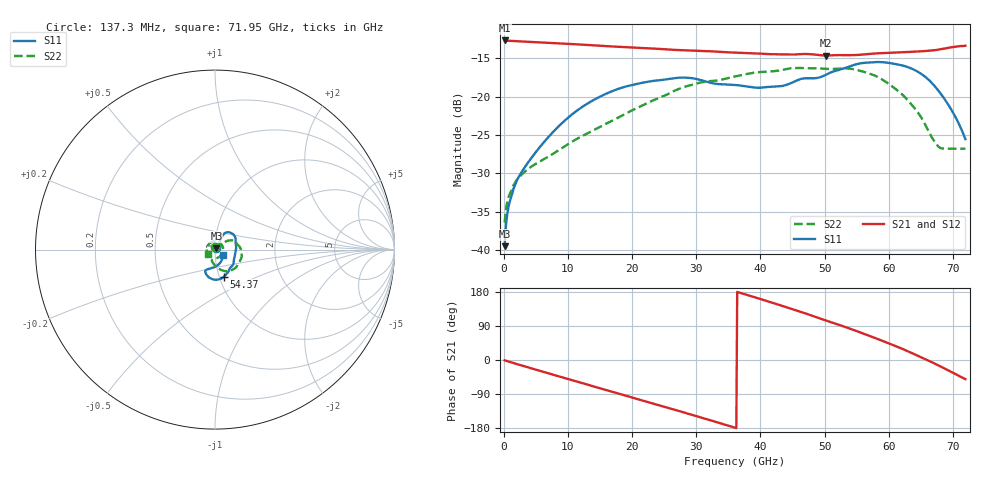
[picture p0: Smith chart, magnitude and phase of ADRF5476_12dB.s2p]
! Device:  ADRF5476
! Description: Flip-Chip, Silicon Digital Step Attenuator
! Frequency:  0.1 GHz -  72 GHz
! Ports:
!  RFC = ATTIN
!  RF1 = ATTOUT
! VDD  =  +3.3 Volts
! VSS  =  -3.3 Volts
! State
! 12dB Attenuation State: D0 = +3.3V, D1 = +3.3V
! Data:  Data was collected using a calibrated network analyzer
!  The reference plane is the package boundry of ADRF5476 switch.
! Notes: Analog Devices supplies this data as a sample of measured data
!  for this product.  Your particular data for this product may vary.
!  Analog Devices reserves the right to change this data at anytime.
# GHZ  S  DB  R  50
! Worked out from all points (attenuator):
!   524 points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, 137.3 MHz to 71.95 GHz, reference 50 ohm
!   highest |S21| = -12.67 dB at 137.3 MHz (marker M1); lowest = -14.6 dB at 50.26 GHz (marker M2)
!   lowest |S11| = -39.5 dB at 137.3 MHz (marker M3), VSWR 1.02, Z = 50.8 + j0.708 ohm
!   |S11| at or under -10 dB: start of sweep to end of sweep
!   |S22| runs from -36.4 to -16.3 dB; largest |S21 - S12| = 0.051
!   S11 on the Smith chart (normalised r, x): 137.3 MHz: 1.02, +0.01; 54.37 GHz: 1.05, -0.33; 71.95 GHz: 1.09, -0.07
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0.1373092  -39.48 41.0  -12.67 -0.9  -12.67 -0.9  -36.40 94.8
0.5492366  -35.29 42.7  -12.70 -3.0  -12.70 -3.0  -33.72 48.4
0.9611641  -33.61 41.9  -12.72 -5.2  -12.72 -5.2  -32.65 38.6
1.785019  -31.42 42.9  -12.76 -9.4  -12.75 -9.4  -31.17 25.0
2.608874  -30.07 44.5  -12.79 -13.5  -12.79 -13.5  -30.29 25.5
7.277386  -24.97 59.2  -12.99 -36.7  -12.98 -36.7  -27.65 32.9
12.22052  -21.34 61.9  -13.22 -61.0  -13.22 -61.0  -25.13 37.1
17.71288  -19.02 57.5  -13.49 -87.8  -13.49 -87.8  -22.79 37.3
24.16641  -17.86 47.1  -13.77 -119.3  -13.76 -119.3  -20.15 31.5
28.69761  -17.53 34.1  -13.96 -141.4  -13.96 -141.4  -18.59 23.0
36.11231  -18.48 8.2  -14.25 -179.0  -14.24 -179.0  -17.35 8.3
43.11508  -18.63 -24.0  -14.48 144.4  -14.48 144.3  -16.56 -8.0
48.05821  -17.60 -49.4  -14.48 116.8  -14.47 116.8  -16.29 -23.0
50.25515  -17.12 -55.7  -14.63 104.0  -14.62 104.0  -16.38 -29.2
54.37443  -15.91 -72.1  -14.58 80.2  -14.57 80.2  -16.40 -44.8
60.0041  -15.59 -93.9  -14.30 44.0  -14.29 43.9  -18.33 -71.4
63.71145  -16.39 -106.7  -14.13 17.5  -14.13 17.4  -21.16 -90.7
66.45763  -17.98 -114.2  -14.00 -3.7  -14.00 -3.4  -24.89 -102.4
67.96803  -19.45 -102.2  -13.83 -16.1  -13.83 -13.4  -26.64 -50.7
68.9292  -20.59 -86.9  -13.69 -24.4  -13.69 -19.1  -26.76 10.6
70.02767  -22.08 -68.6  -13.52 -33.9  -13.52 -25.6  -26.77 83.9
71.95  -25.53 -36.5  -13.35 -50.5  -13.35 -36.9  -26.78 -147.8
